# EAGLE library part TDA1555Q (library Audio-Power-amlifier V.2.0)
The TDA1555Q contains four identical amplifiers with differential input stages (two inverting and two non-inverting) and can be used for single-ended or bridge applications. The gain of each amplifier is fixed at 20 dB (26 dB in BTL). Special features of this device are:
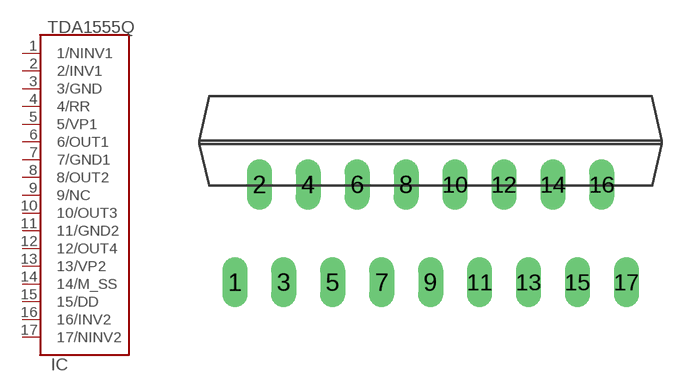
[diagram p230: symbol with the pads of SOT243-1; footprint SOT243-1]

Designator prefix IC

## TDA1555Q  [SOT243-1]
1  1/NINV1  in
2  2/INV1  in
3  3/GND  pwr
4  4/RR  in
5  5/VP1  pwr
6  6/OUT1  out
7  7/GND1  pwr
8  8/OUT2  out
9  9/NC  nc
10  10/OUT3  out
11  11/GND2  pwr
12  12/OUT4  out
13  13/VP2  pwr
14  14/M_SS  in
15  15/DD  in
16  16/INV2  in
17  17/NINV2  in

## Footprint SOT243-1 (pad centres in mm)
DBS17P: plastic DIL-bent-SIL power package; 17 leads (lead length 7.7 mm)
drill 0.8 long: 1 -10.16,-5.08; 2 -8.89,0; 3 -7.62,-5.08; 4 -6.35,0; 5 -5.08,-5.08; 6 -3.81,0; 7 -2.54,-5.08; 8 -1.27,0; 9 0,-5.08; 10 1.27,0; 11 2.54,-5.08; 12 3.81,0; 13 5.08,-5.08; 14 6.35,0; 15 7.62,-5.08; 16 8.89,0; 17 10.17,-5.08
